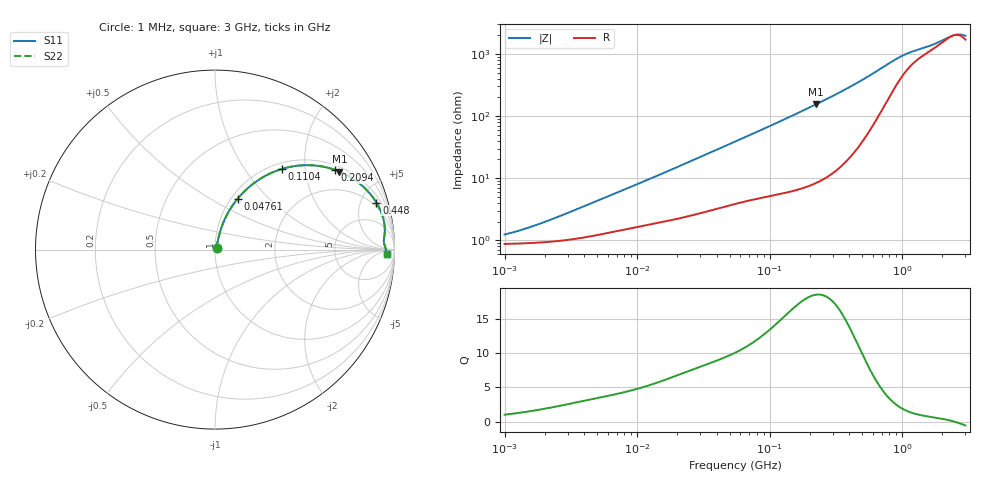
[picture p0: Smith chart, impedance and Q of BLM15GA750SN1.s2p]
! BLM15GA750SN1
# Hz S RI R 50
!Freq.(Hz) S11(Real) S11(Imag) S21(Real) S21(Imag) S12(Real) S12(Imag) S22(Real) S22(Imag)
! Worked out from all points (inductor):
!   401 points, 1 MHz to 3 GHz, reference 50 ohm
!   read as one part in series: L = 132 nH near 3.979 MHz
!   highest Q = 18.5 at 222.4 MHz (marker M1), where L = 110 nH
!   self-resonance near 2.456 GHz
!   S11 on the Smith chart (normalised r, x): 1 MHz: 1.02, +0.02; 47.61 MHz: 1.07, +0.68; 110.4 MHz: 1.11, +1.51; 209.4 MHz: 1.16, +2.88; 448 MHz: 1.56, +6.67; 3 GHz: 35, -20
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1000000  0.0087 0.00857  0.9913 -0.00857  0.9913 -0.00857  0.0087 0.00857
1716745  0.00922 0.0146  0.9908 -0.0146  0.9908 -0.0146  0.00922 0.0146
3823119  0.0118 0.0315  0.9882 -0.0315  0.9882 -0.0315  0.0118 0.0315
8017732  0.0185 0.0617  0.9815 -0.0617  0.9815 -0.0617  0.0185 0.0617
1.461624e7  0.0303 0.1055  0.9697 -0.1055  0.9697 -0.1055  0.0303 0.1055
2.829425e7  0.0635 0.1883  0.9365 -0.1883  0.9365 -0.1883  0.0635 0.1883
4.761141e7  0.1271 0.2846  0.8729 -0.2846  0.8729 -0.2846  0.1271 0.2846
5.477226e7  0.1536 0.3143  0.8464 -0.3143  0.8464 -0.3143  0.1536 0.3143
7.852918e7  0.2473 0.3913  0.7527 -0.3913  0.7527 -0.3913  0.2473 0.3913
1.103592e8  0.3739 0.4498  0.6261 -0.4498  0.6261 -0.4498  0.3739 0.4498
1.520175e8  0.5195 0.4705  0.4805 -0.4705  0.4805 -0.4705  0.5195 0.4705
2.094008e8  0.6675 0.4447  0.3325 -0.4447  0.3325 -0.4447  0.6675 0.4447
2.223601e8  0.6932 0.435  0.3068 -0.435  0.3068 -0.435  0.6932 0.435
3.188066e8  0.8224 0.3538  0.1776 -0.3538  0.1776 -0.3538  0.8224 0.3538
4.480278e8  0.8995 0.2614  0.1005 -0.2614  0.1005 -0.2614  0.8995 0.2614
5.929311e8  0.9331 0.1885  0.0669 -0.1885  0.0669 -0.1885  0.9331 0.1885
8.005644e8  0.9459 0.1222  0.0541 -0.1222  0.0541 -0.1222  0.9459 0.1222
1.080907e9  0.9435 0.0746  0.0565 -0.0746  0.0565 -0.0746  0.9435 0.0746
1.67892e9  0.9421 0.0345  0.0579 -0.0345  0.0579 -0.0345  0.9421 0.0345
2.359433e9  0.9514 0.00425  0.0486 -0.00425  0.0486 -0.00425  0.9514 0.00425
2.660507e9  0.9547 -0.00889  0.0453 0.00889  0.0453 0.00889  0.9547 -0.00889
3e9  0.9572 -0.0233  0.0428 0.0233  0.0428 0.0233  0.9572 -0.0233
